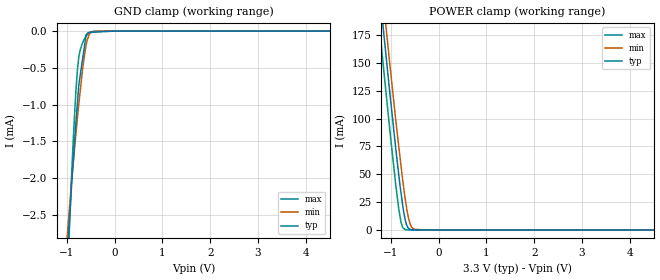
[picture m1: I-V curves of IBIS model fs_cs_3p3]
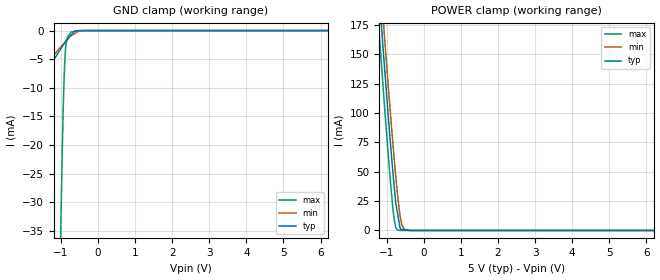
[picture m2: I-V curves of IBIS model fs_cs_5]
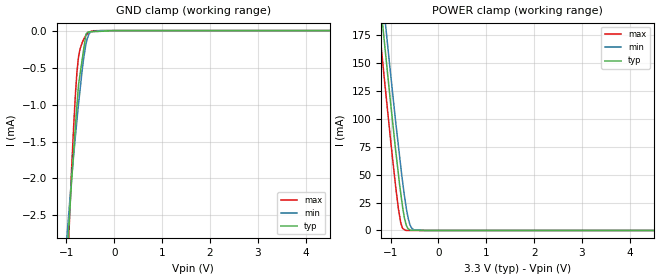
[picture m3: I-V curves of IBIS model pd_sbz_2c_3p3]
|Texas Instruments Incorporated
| 18-Bit 600KSPS Serial ADC with Ref and Unipolar Pseudo Diff Input
| Marketing part#   Digital Voltage Range   Package-type   #pins
| ADS8380IBRHPR   2.7v - 5.25v   VQFN   28
| ADS8380IBRHPRG4   2.7v - 5.25v   VQFN   28
| ADS8380IBRHPT   2.7v - 5.25v   VQFN   28
| ADS8380IBRHPTG4   2.7v - 5.25v   VQFN   28
| ADS8380IRHPR   2.7v - 5.25v   VQFN   28
| ADS8380IRHPRG4   2.7v - 5.25v   VQFN   28
| ADS8380IRHPT   2.7v - 5.25v   VQFN   28
| ADS8380IRHPTG4   2.7v - 5.25v   VQFN   28
[IBIS Ver]   3.2
[File name]   ads8380.ibs
|SIMDE Ver   V3.0 - 201101 - Build 457
[File Rev]   1.0
[Date]   5/18/2011
[Source]
| Texas Instruments Incorporated.
| Analog-eLab Design Center, HPA
| 12500 TI Blvd
| Dallas, TX -75243
| e-mail: elab_ibis@list.ti.com
[Notes]   Revision History:
| Rev 1.0: 5/18/2011
| - Initial version of the model
| - Model generated from simulations in TISPICE
| - Model matched to SPICE simulation
| - C_comp although listed in numerical order of value are
|   obtained from varying PVT conditions. For PVT conditions for
|   each specific value refer the buffer description under
|   respective [Model]. IBIS model user is responsible for using
|   appropriate C_comp to simulate for Signal Integrity.
| - Model names with a trailing _3p3 contains the model for
|   3.3V [3.0V and 3.6V]. Model names with a trailing _5 contains
|   the model for 5.0V [4.75V and 5.25V].
| - SDO pin ibis is modeled in two modes of operation sdo_1drv_*
|   with single driver & sdo_2drv_* 2 driver blocks connected to SDO pad pin.
|   Inbuilt OR logic is used for mode selection.
[Disclaimer]
| This model is designed as an aid for customers of Texas Instruments.
| TI and its licensors and suppliers make no warranties, either expressed
| or implied, with respect to this  model, including the warranties of
| merchantability or fitness for a particular purpose. The model is
| provided solely on an "as is" basis. The entire risk as to its quality
| and performance is with the customer.
[Copyright]
 (C) Copyright 2011 Texas Instruments Incorporated.All rights reserved.
|   ADS8380RHP
[Component]   ADS8380RHP
[Manufacturer]   TI
[Package]   |28 VQFN - RHP package
|   typ   min   max
R_pkg   0.00007   0.00007   0.00007
L_pkg   0.00128nH   0.00128nH   0.00128nH
C_pkg   0.12198pF   0.12021pF   0.12296pF
[Pin]  signal_name   model_name   R_pin   L_pin   C_pin
1   _SB/2C   pd_sbz_2c   0.00007   0.00128nH  0.12251pF
2   AGND   GND   0.00007   0.00128nH  0.12249pF
3   +VA   POWER   0.00007   0.00128nH  0.12268pF
4   AGND   GND   0.00007   0.00128nH  0.12271pF
5   AGND   GND   0.00007   0.00128nH  0.12269pF
6   +VA   POWER   0.00007   0.00128nH  0.12262pF
7   REFM   GND   0.00007   0.00128nH  0.12264pF
8   REFIN   TERM   0.00007   0.00128nH  0.12021pF
9   REFOUT   TERM   0.00007   0.00128nH  0.12025pF
10   NC   NC   0.00007   0.00128nH  0.12029pF
11   +IN   TERM   0.00007   0.00128nH  0.12033pF
12   -IN   TERM   0.00007   0.00128nH  0.12027pF
13   NC   NC   0.00007   0.00128nH  0.12029pF
14   +VA   POWER   0.00007   0.00128nH  0.12018pF
15   AGND   GND   0.00007   0.00128nH  0.12012pF
16   +VA   POWER   0.00007   0.00128nH  0.12017pF
17   +VA   POWER   0.00007   0.00128nH  0.12030pF
18   AGND   GND   0.00007   0.00128nH  0.12030pF
19   AGND   GND   0.00007   0.00128nH  0.12022pF
20   +VBD   POWER   0.00007   0.00128nH  0.12021pF
21   BDGND   GND   0.00007   0.00128nH  0.12023pF
22   BUSY   busy   0.00007   0.00128nH  0.12287pF
23   SDO   sdo   0.00007   0.00128nH  0.12289pF
24   SCLK   sclk_convest   0.00007   0.00128nH  0.12285pF
25   _CONVST   sclk_convest   0.00007   0.00128nH  0.12296pF
26   _CS   fs_cs   0.00007   0.00128nH  0.12296pF
27   FS   fs_cs   0.00007   0.00128nH  0.12285pF
28   PD   pd_sbz_2c   0.00007   0.00128nH  0.12285pF
|   Model Selectors
[Model Selector] fs_cs
fs_cs_3p3  3.3V  digital input
fs_cs_5   5.0V  digital input
[Model Selector] pd_sbz_2c
pd_sbz_2c_3p3  3.3V  digital input
pd_sbz_2c_5   5.0V  digital input
[Model Selector] sclk_convest
sclk_convest_3p3  3.3V digital input
sclk_convest_5   5.0V digital input
[Model Selector] busy
busy_3p3  3.3V  digital 3-state
busy_5   5.0V  digital 3-state
[Model Selector] sdo
sdo_1drv_3p3  3.3V  digital 3-state
sdo_1drv_5   5.0V  digital 3-state
sdo_2drv_3p3  3.3V  digital 3-state
sdo_2drv_5   5.0V  digital 3-state
[Model Selector] TERM
TERM_3p3  3.3V nominal termination
TERM_5   5.0V nominal termination
[Model] TERM_3p3
Model_type Terminator
C_comp   1.0e-20F  1.0e-20F  1.0e-20F
|   typ   min   max
[Voltage Range]   3.3V   3.0V   3.6V
[POWER Clamp Reference]   3.3V   3.0V   3.6V
[GND Clamp Reference]   0V   0V   0V
|Ambient Temperature   25   85   -40
|Junction Temperature
[Temperature Range]   35   95   -40
[Model] TERM_5
Model_type Terminator
C_comp   1.0e-20F  1.0e-20F  1.0e-20F
|   typ   min   max
[Voltage Range]   5.0V   4.75V   5.25V
[POWER Clamp Reference]   5.0V   4.75V   5.25V
[GND Clamp Reference]   0V   0V   0V
|Ambient Temperature   25   85   -40
|Junction Temperature
[Temperature Range]   35   95   -40
| Models and submodels in the file (14): fs_cs_3p3 (Input), fs_cs_5 (Input), pd_sbz_2c_3p3 (Input), pd_sbz_2c_5 (Input), sclk_convest_3p3 (Input), sclk_convest_5 (Input), busy_3p3 (3-state), busy_5 (3-state), sdo_1drv_3p3 (3-state), sdo_1drv_5 (3-state), sdo_2drv_3p3 (3-state), sdo_2drv_5 (3-state), TERM_3p3 (Terminator), TERM_5 (Terminator)
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|   fs_cs_3p3 Model
[Model]   fs_cs_3p3
Model_type   Input
Vinl = 0.8
Vinh = 2.3
|   typ   min   max
|   (nom PVT)   (fast PVT)   (slow PVT)
|C_comp from frequency sweep method (F=40MHz)
|Average
C_comp   9.345e-13   8.948e-13   9.802e-13
|C_comp from LC tank measurement(L=1nH)
|Average
|Resonant Frequency(Hz)   6.530e+09   6.860e+09   6.210e+09
|C_comp   5.946e-13   5.388e-13   6.575e-13
| Where nom  PVT is Nominal Process, 3.3V, 35C
|   Fast PVT is Strong Process,  3.6V, -40C
|   Slow PVT is Weak Process,   3V, 95C
[Model Spec]
Vinl   0.8   0.8   0.8
Vinh   2.3   2.0   2.6
[Voltage Range]   3.3   3   3.6
|Ambient Temperature   25   85   -40
|Junction Temperature
[Temperature Range]   35   95   -40
[Power Clamp Reference]   3.3   3   3.6
[GND Clamp Reference]   0   0   0
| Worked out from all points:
|   GND clamp passes 1 mA (typ) near -0.78 V on its own axis
|   POWER clamp passes 1 mA (typ) near -0.61 V on its own axis
[GND Clamp]
|   Voltage   I(typ)   I(min)   I(max)
-3.3V     -29.5mA    -22.08mA   -346.9mA
-1.48V    -8.435mA   -6.749mA   -11.2mA
-897.6mV  -2.079mA   -2.033mA   -1.938mA
-813.6mV  -1.291mA   -1.432mA   -869.3uA
-781.2mV  -1.016mA   -1.213mA   -563uA
-752.4mV  -772.5uA   -1.02mA    -377.4uA
-666mV    -368uA     -504.3uA   -154.1uA
-594mV    -49.28uA   -188.5uA   -63.98uA
-547.8mV  -18.81uA   -78.25uA   -34.03uA
-483mV    -16.57uA   -13.84uA   -10.13uA
-285mV    -9.73uA    -61.45nA   -1.03uA
6.6V      0A         0A         0A
[POWER Clamp]
|   Voltage   I(typ)   I(min)   I(max)
-3.3V     1.135A     1.155A     1.11A
-1.318V   249.1mA    274.8mA    216.8mA
-1.176V   187.9mA    213.6mA    155.3mA
-1.13V    168.7mA    194.3mA    135.5mA
-1.023V   123.4mA    149.3mA    90.46mA
-896.4mV  72.45mA    98.1mA     40mA
-835.2mV  49.7mA     75.13mA    19.03mA
-784.8mV  32.38mA    56.22mA    6.372mA
-691.2mV  7.748mA    25.44mA    159.7uA
-597mV    508.4uA    5.363mA    2.122uA
-516mV    127uA      660uA      747.1nA
6.6V      0A         0A         0A
|   fs_cs_5 Model
[Model]   fs_cs_5
Model_type   Input
Vinl = 0.8
Vinh = 4.0
|   typ   min   max
|   (nom PVT)   (fast PVT)   (slow PVT)
|C_comp from frequency sweep method (F=40MHz)
|Average
C_comp   9.085e-13   8.893e-13   9.134e-13
|C_comp from LC tank measurement(L=1nH)
|Average
|Resonant Frequency(Hz)   6.870e+09   7.150e+09   6.610e+09
|C_comp   5.372e-13   4.960e-13   5.803e-13
| Where nom  PVT is Nominal Process, 5V, 35C
|   Fast PVT is Strong Process,  5.25V, -40C
|   Slow PVT is Weak Process,   4.75V, 95C
[Model Spec]
Vinl   0.8   0.8   0.8
Vinh   4.0   3.75   4.25
[Voltage Range]   5   4.75   5.25
|Ambient Temperature   25   85   -40
|Junction Temperature
[Temperature Range]   35   95   -40
[Power Clamp Reference]   5   4.75   5.25
[GND Clamp Reference]   0   0   0
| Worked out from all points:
|   GND clamp passes 1 mA (typ) near -0.76 V on its own axis
|   POWER clamp passes 1 mA (typ) near -0.62 V on its own axis
[GND Clamp]
|   Voltage   I(typ)   I(min)   I(max)
-5V       -51.14mA   -37.96mA   -1.888A
-4.75V    -47.95mA   -35.65mA   -1.771A
-4.21V    -41.13mA   -30.65mA   -1.516A
-3.533V   -32.56mA   -24.38mA   -1.198A
-2.67V    -21.64mA   -16.53mA   -792.8mA
-1.008V   -3.206mA   -2.891mA   -36.15mA
-939.7mV  -2.519mA   -2.392mA   -14.05mA
-892.5mV  -2.043mA   -2.046mA   -4.874mA
-829.5mV  -1.508mA   -1.585mA   -1.265mA
-729.8mV  -784.8uA   -924.3uA   -289.8uA
-503.5mV  -20.08uA   -23.98uA   -21.48uA
10V       0A         0A         0A
[POWER Clamp]
|   Voltage   I(typ)   I(min)   I(max)
-5V       1.905A     1.922A     1.884A
-1.302V   242mA      267.3mA    209.7mA
-1.126V   166.8mA    192.3mA    134.1mA
-1.08V    147.2mA    173.1mA    114.4mA
-955.5mV  95.9mA     121.9mA    62.77mA
-834.7mV  49.93mA    74.38mA    18.9mA
-761.2mV  24.49mA    47.49mA    2.961mA
-698.3mV  12.62mA    27.18mA    218.3uA
-640mV    1.834mA    12.45mA    14.73uA
-598.5mV  870.6uA    5.545mA    1.881uA
-356.3mV  494.1nA    6.232uA    1.12uA
10V       0A         0A         0A
|   pd_sbz_2c_3p3 Model
[Model]   pd_sbz_2c_3p3
Model_type   Input
Vinl = 0.8
Vinh = 2.3
|   typ   min   max
|   (nom PVT)   (fast PVT)   (slow PVT)
|C_comp from frequency sweep method (F=40MHz)
|Average
C_comp   9.314e-13   9.057e-13   9.837e-13
|C_comp from LC tank measurement(L=1nH)
|Average
|Resonant Frequency(Hz)   6.540e+09   6.860e+09   6.220e+09
|C_comp   5.928e-13   5.388e-13   6.554e-13
| Where nom  PVT is Nominal Process, 3.3V, 35C
|   Fast PVT is Strong Process,  3.6V, -40C
|   Slow PVT is Weak Process,   3V, 95C
[Model Spec]
Vinl   0.8   0.8   0.8
Vinh   2.3   2.0   2.6
[Voltage Range]   3.3   3   3.6
|Ambient Temperature   25   85   -40
|Junction Temperature
[Temperature Range]   35   95   -40
[Power Clamp Reference]   3.3   3   3.6
[GND Clamp Reference]   0   0   0
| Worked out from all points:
|   GND clamp passes 1 mA (typ) near -0.78 V on its own axis
|   POWER clamp passes 1 mA (typ) near -0.61 V on its own axis
[GND Clamp]
|   Voltage   I(typ)   I(min)   I(max)
-3.3V     -29.5mA    -22.08mA   -346.9mA
-1.48V    -8.435mA   -6.749mA   -11.2mA
-897.6mV  -2.079mA   -2.033mA   -1.938mA
-813.6mV  -1.291mA   -1.432mA   -869.3uA
-781.2mV  -1.016mA   -1.213mA   -563uA
-752.4mV  -772.5uA   -1.02mA    -377.4uA
-666mV    -368uA     -504.3uA   -154.1uA
-594mV    -49.28uA   -188.5uA   -63.98uA
-547.8mV  -18.81uA   -78.25uA   -34.03uA
-483mV    -16.57uA   -13.84uA   -10.13uA
-285mV    -9.73uA    -61.45nA   -1.03uA
6.6V      0A         0A         0A
[POWER Clamp]
|   Voltage   I(typ)   I(min)   I(max)
-3.3V     1.135A     1.155A     1.11A
-1.318V   249.1mA    274.8mA    216.8mA
-1.176V   187.9mA    213.6mA    155.3mA
-1.13V    168.7mA    194.3mA    135.5mA
-1.023V   123.4mA    149.3mA    90.46mA
-896.4mV  72.45mA    98.1mA     40mA
-835.2mV  49.7mA     75.13mA    19.03mA
-784.8mV  32.38mA    56.22mA    6.372mA
-691.2mV  7.748mA    25.44mA    159.7uA
-597mV    508.4uA    5.363mA    2.122uA
-516mV    127uA      660uA      747.1nA
6.6V      0A         0A         0A
